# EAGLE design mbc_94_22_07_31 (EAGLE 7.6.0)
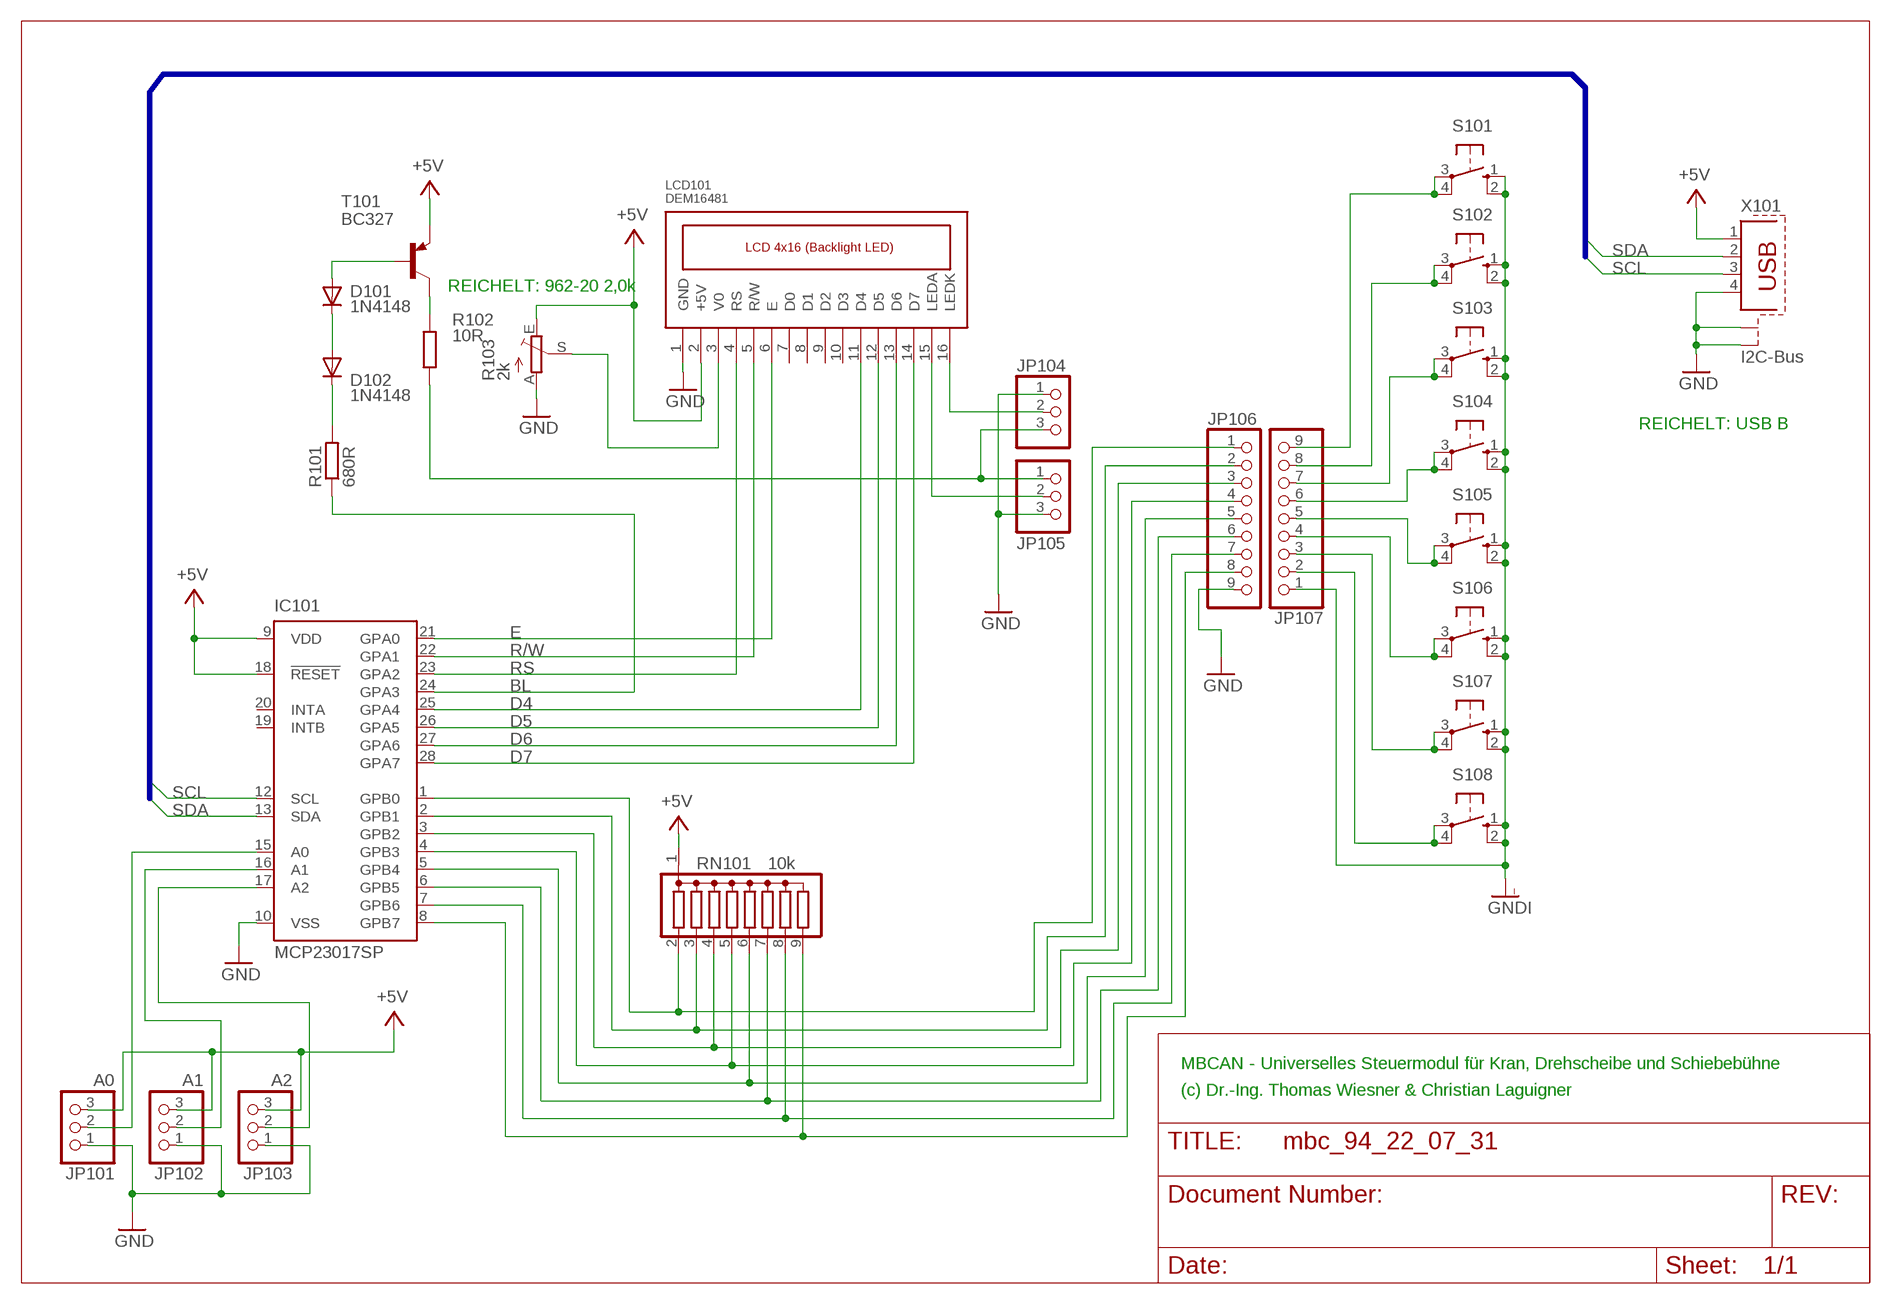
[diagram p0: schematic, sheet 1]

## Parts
D101  1N4148  1N4148DO35-10  [DO35-10]
D102  1N4148  1N4148DO35-10  [DO35-10]
IC101  MCP23017SP  [DIL28-3]
JP101  A0  PINHD-1X3  [1X03]
JP102  A1  PINHD-1X3  [1X03]
JP103  A2  PINHD-1X3  [1X03]
JP104  PINHD-1X3  [1X03]
JP105  PINHD-1X3  [1X03]
JP106  PINHD-1X9  [1X09]
JP107  PINHD-1X9  [1X09]
LCD101  DEM16481  [LCD4X16]
R101  680R  R-EU_0207/10  [0207/10]
R102  10R  R-EU_0207/10  [0207/10]
R103  2k  TRIM_EU-S43P  [SP19L]
RN101  10k  G08R  [SIL9]
S101  10-XX  [B3F-10XX]
S102  10-XX  [B3F-10XX]
S103  10-XX  [B3F-10XX]
S104  10-XX  [B3F-10XX]
S105  10-XX  [B3F-10XX]
S106  10-XX  [B3F-10XX]
S107  10-XX  [B3F-10XX]
S108  10-XX  [B3F-10XX]
T101  BC327  -PNP-TO92  [TO92]
X101  I2C-Bus  PN61729-S  [PN61729-S]

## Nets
+5V: IC101.9(VDD) IC101.18(!RESET) JP101.3 JP102.3 JP103.3 LCD101.2(+5V) R103.E RN101.1 T101.1(E) X101.1
BL: IC101.24(GPA3) R101.1
D4: IC101.25(GPA4) LCD101.11(D4)
D5: IC101.26(GPA5) LCD101.12(D5)
D6: IC101.27(GPA6) LCD101.13(D6)
D7: IC101.28(GPA7) LCD101.14(D7)
E: IC101.21(GPA0) LCD101.6(E)
GND: IC101.10(VSS) JP101.1 JP102.1 JP103.1 JP104.1 JP105.3 JP106.9 LCD101.1(GND) R103.A X101.4 X101.S1 X101.S2
GNDI: JP107.1 S101.1(S) S101.2(S1) S102.1(S) S102.2(S1) S103.1(S) S103.2(S1) S104.1(S) S104.2(S1) S105.1(S) S105.2(S1) S106.1(S) S106.2(S1) S107.1(S) S107.2(S1) S108.1(S) S108.2(S1)
N$1: IC101.1(GPB0) JP106.1 RN101.2
N$2: IC101.2(GPB1) JP106.2 RN101.3
N$3: IC101.3(GPB2) JP106.3 RN101.4
N$4: IC101.4(GPB3) JP106.4 RN101.5
N$5: IC101.5(GPB4) JP106.5 RN101.6
N$6: IC101.6(GPB5) JP106.6 RN101.7
N$7: IC101.7(GPB6) JP106.7 RN101.8
N$8: IC101.8(GPB7) JP106.8 RN101.9
N$11: JP105.2 LCD101.15(LEDA)
N$12: JP104.2 LCD101.16(LEDK)
N$14: JP107.9 S101.3(P) S101.4(P1)
N$15: JP107.8 S102.3(P) S102.4(P1)
N$16: JP107.7 S103.3(P) S103.4(P1)
N$17: JP107.6 S104.3(P) S104.4(P1)
N$18: JP107.5 S105.3(P) S105.4(P1)
N$19: JP107.4 S106.3(P) S106.4(P1)
N$20: JP107.3 S107.3(P) S107.4(P1)
N$21: JP107.2 S108.3(P) S108.4(P1)
N$22: IC101.15(A0) JP101.2
N$23: IC101.16(A1) JP102.2
N$24: LCD101.3(V0) R103.S
N$25: D102.C R101.2
N$26: D101.C D102.A
N$27: D101.A T101.2(B)
N$28: R102.2 T101.3(C)
N$29: IC101.17(A2) JP103.2
N$35: JP104.3 JP105.1 R102.1
R/W: IC101.22(GPA1) LCD101.5(R/W)
RS: IC101.23(GPA2) LCD101.4(RS)
SCL: IC101.12(SCL) X101.3
SDA: IC101.13(SDA) X101.2
Unconnected: IC101.19(INTB) IC101.20(INTA) LCD101.7(D0) LCD101.8(D1) LCD101.9(D2) LCD101.10(D3)

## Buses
B$3

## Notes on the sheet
- REICHELT: 962-20 2,0k
- REICHELT: USB B
- MBCAN - Universelles Steuermodul für Kran, Drehscheibe und Schiebebühne
- (c) Dr.-Ing. Thomas Wiesner & Christian Laguigner

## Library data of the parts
D101 D102 = diode:1N4148: DIODE
IC101 = microchip:MCP23017: http://ww1.microchip.com/downloads/en/DeviceDoc/21952a.pdf Source: http://ww1.microchip.com/downloads/en/DeviceDoc/21952a.pdf; MF: MICROCHIP; MPN: MCP23017-E/SP; OC_FARNELL: 1332088; OC_NEWARK: 31K2959
JP101-JP105 = pinhead:PINHD-1X3: PIN HEADER
JP106 JP107 = pinhead:PINHD-1X9: PIN HEADER
LCD101 = mbc:DEM16481
R101 R102 = resistor:R-EU_: RESISTOR, European symbol
R103 = pot:TRIM_EU-: POTENTIOMETER
RN101 = resistor-sil:G08R: SIL RESISTOR; OC_FARNELL: unknown; OC_NEWARK: unknown
S101-S108 = switch-omron:10-XX: OMRON SWITCH; MPN: B3F-1000; OC_FARNELL: 176432; OC_NEWARK: 36M3542
T101 = transistor:*-PNP-: PNP Transistror
X101 = con-berg:PN61729-S: BERG USB connector; OC_FARNELL: unknown; OC_NEWARK: unknown

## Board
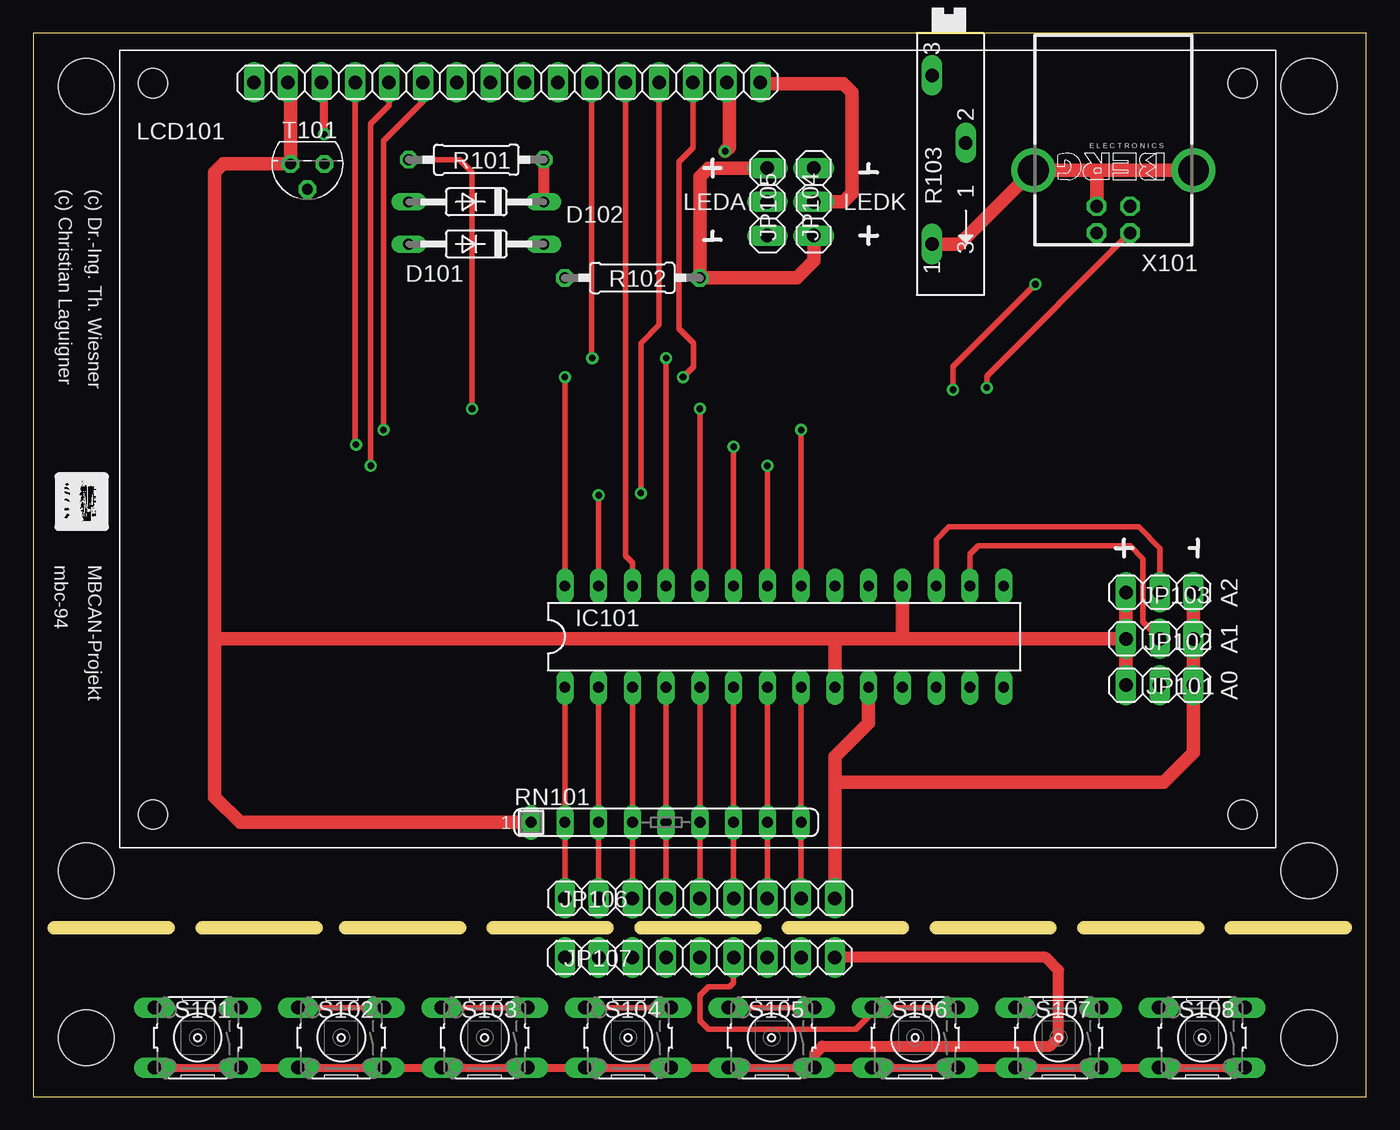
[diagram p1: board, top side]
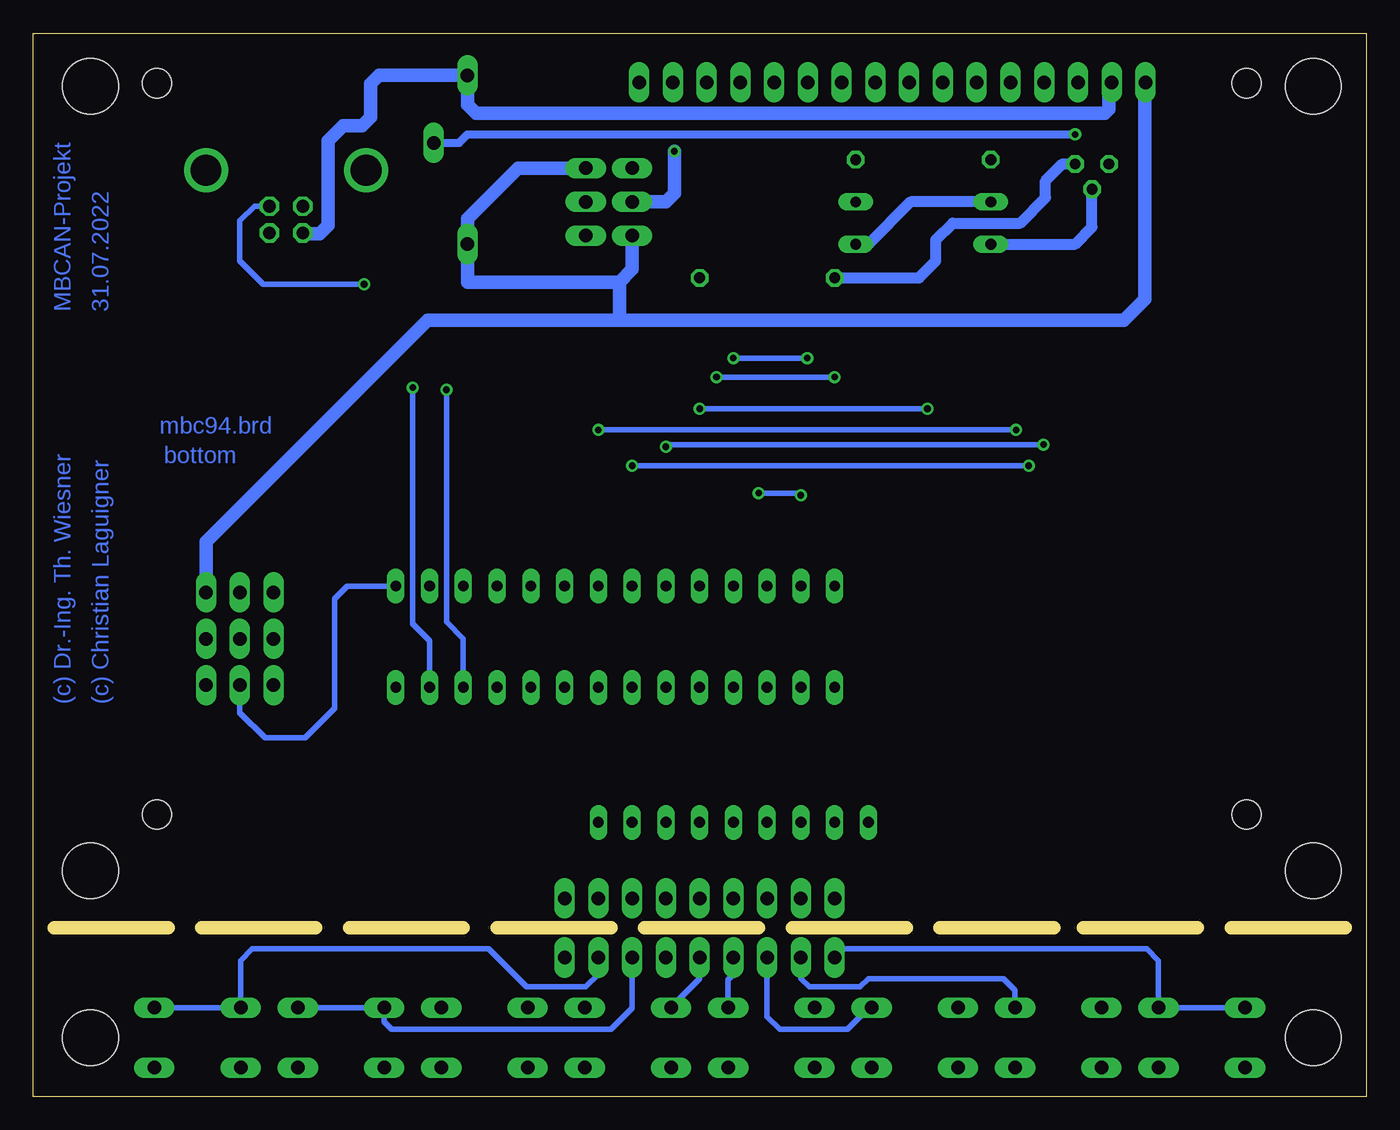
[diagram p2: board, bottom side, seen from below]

Size 100.31 x 80 mm. Coordinates in mm from the lower left corner, seen from the top.
Outline: 0,0 100.31,0 100.31,80 0,80 0,0
Copper layers (1*16): Top 0.035mm / dielectric 1.5mm / Bottom 0.035mm
Design rules "default *": minimum track width 10mil, minimum drill 0.5mm, track to track 8mil, track to pad 8mil, pad to pad 8mil, via to via 8mil, smd to smd 8mil, copper to edge 40mil, drill to drill 8mil, minimum pad ring 10mil, minimum via ring 8mil, stop-mask expansion 4mil, vias tented up to drill 0mil, thermal gap 10mil
Holes 4.2 mm at 4,76 96,76 4,4.45 96,4.45 4,17 96,17
Milling: 9 lines

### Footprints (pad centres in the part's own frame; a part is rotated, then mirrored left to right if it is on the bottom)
DO35-10 = drill 0.813 long: A 5.08,0; C -5.08,0
DIL28-3 = drill 0.813 long: 1 -16.51,-3.81; 2 -13.97,-3.81; 3 -11.43,-3.81; 4 -8.89,-3.81; 5 -6.35,-3.81; 6 -3.81,-3.81; 7 -1.27,-3.81; 8 1.27,-3.81; 9 3.81,-3.81; 10 6.35,-3.81; 11 8.89,-3.81; 12 11.43,-3.81; 13 13.97,-3.81; 14 16.51,-3.81; 15 16.51,3.81; 16 13.97,3.81; 17 11.43,3.81; 18 8.89,3.81; 19 6.35,3.81; 20 3.81,3.81; 21 1.27,3.81; 22 -1.27,3.81; 23 -3.81,3.81; 24 -6.35,3.81; 25 -8.89,3.81; 26 -11.43,3.81; 27 -13.97,3.81; 28 -16.51,3.81
1X03 = drill 1.016 long: 1 -2.54,0; 2 0,0; 3 2.54,0
1X09 = drill 1.016 long: 1 -10.16,0; 2 -7.62,0; 3 -5.08,0; 4 -2.54,0; 5 0,0; 6 2.54,0; 7 5.08,0; 8 7.62,0; 9 10.16,0
LCD4X16 = drill 1.016 long: 1 10.11,57.57; 2 12.65,57.57; 3 15.19,57.57; 4 17.73,57.57; 5 20.27,57.57; 6 22.81,57.57; 7 25.35,57.57; 8 27.89,57.57; 9 30.43,57.57; 10 32.97,57.57; 11 35.51,57.57; 12 38.05,57.57; 13 40.59,57.57; 14 43.13,57.57; 15 45.67,57.57; 16 48.21,57.57 | hole 2.2: 2.5,2.5; 2.5,57.5; 84.5,57.5; 84.5,2.5
0207/10 = drill 0.813 octagon: 1 -5.08,0; 2 5.08,0
SP19L = drill 1.016 long: A 5.715,-1.27; E -6.985,-1.27; S -1.905,1.27
SIL9 = drill 0.813 long: 1 -10.16,0; 2 -7.62,0; 3 -5.08,0; 4 -2.54,0; 5 0,0; 6 2.54,0; 7 5.08,0; 8 7.62,0; 9 10.16,0
B3F-10XX = drill 1.016 long: 1 -3.251,2.261; 2 3.251,2.261; 3 -3.251,-2.261; 4 3.251,-2.261
TO92 = drill 0.813 octagon: 1 1.27,0; 2 0,1.905; 3 -1.27,0
PN61729-S = drill 0.95 octagon: 1 1.25,4.71; 2 -1.25,4.71; 3 -1.25,2.71; 4 1.25,2.71 | drill 2.3 pad 2.9: S1 -6.02,0; S2 6.02,0

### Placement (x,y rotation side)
D101  33.34,64.14 180 top
D102  33.34,67.31 180 top
IC101  56.52,34.61 0 top
JP101  84.77,30.96 180 top
JP102  84.77,34.45 180 top
JP103  84.77,37.94 180 top
JP104  58.74,67.31 270 top
JP105  55.24,67.31 270 top
JP106  50.16,14.92 0 top
JP107  50.16,10.48 180 top
LCD101  6.51,18.73 0 top
R101  33.34,70.48 0 top
R102  45.09,61.59 180 top
R103  68.9,69.85 270 top
RN101  47.62,20.64 0 top
S101  12.38,4.45 180 top
S102  23.18,4.45 180 top
S103  33.97,4.45 180 top
S104  44.77,4.45 180 top
S105  55.56,4.45 180 top
S106  66.36,4.45 180 top
S107  77.15,4.45 180 top
S108  87.95,4.45 180 top
T101  20.64,70.17 180 top
X101  81.28,69.69 180 top

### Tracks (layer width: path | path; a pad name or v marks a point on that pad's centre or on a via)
+5V
  Top 1.016: RN101.1 15.56,20.64 13.65,22.54 13.65,34.45 | 13.65,34.45 13.65,69.53 14.29,70.17 T101.1 19.37,76.25 LCD101.2 | IC101.9 60.33,34.45 | 60.33,34.45 13.65,34.45 | 60.33,34.45 65.41,34.45 | JP103.3 JP102.3 | JP102.3 JP101.3 | IC101.18 65.41,34.45 | 65.41,34.45 JP102.3
  Bottom 1.016: LCD101.2 19.37,76.25 19.37,74.3 19.68,73.98 66.99,73.98 67.63,74.61 R103.E 74.3,76.83 74.93,76.2 74.93,73.66 75.56,73.03 76.99,73.03 78.11,71.91 78.11,65.56 78.74,64.93 79.98,64.93 X101.1
BL  (via drill 0.5)
  Top 0.406: v33.02,51.75 33.02,69.53 32.07,70.48 R101.1 | v50.16,51.75 IC101.24
  Bottom 0.406: v33.02,51.75 v50.16,51.75
D4  (via drill 0.5)
  Top 0.406: LCD101.11 42.02,55.61 v42.07,55.56 | v47.62,55.56 IC101.25
  Bottom 0.406: v42.07,55.56 v47.62,55.56
D5
  Top 0.406: LCD101.12 44.56,40.69 45.09,40.16 IC101.26
D6  (via drill 0.5)
  Top 0.406: LCD101.13 47.1,58.05 45.72,56.67 v45.72,45.4 | v42.55,45.24 IC101.27
  Bottom 0.406: v45.72,45.4 42.7,45.4 v42.55,45.24
D7  (via drill 0.5)
  Top 0.406: LCD101.14 49.64,71.39 48.58,70.33 48.58,57.78 49.69,56.67 49.69,54.93 v48.9,54.13 | v40.01,54.13 IC101.28
  Bottom 0.406: v48.9,54.13 v40.01,54.13
E  (via drill 0.5)
  Top 0.406: LCD101.6 29.32,74.88 26.35,71.91 v26.35,50.16 | v57.78,50.16 IC101.21
  Bottom 0.406: v26.35,50.16 v57.78,50.16
GND
  Top 1.016: X101.S1 80.17,69.69 | 80.17,69.69 X101.S2 75.25,69.69 69.69,64.14 R103.A | X101.4 80.03,69.55 80.17,69.69 | JP106.9 60.33,23.65 | 60.33,23.65 60.33,25.56 62.87,28.1 IC101.10 | JP103.1 JP102.1 JP101.1 87.31,25.88 85.09,23.65 60.33,23.65
  Bottom 1.016: LCD101.1 16.68,76.2 16.68,60 18.26,58.42 56.2,58.42 | JP104.1 63.82,69.85 67.63,66.04 R103.A 67.63,61.28 56.2,61.28 | JP105.3 55.24,62.23 56.2,61.28 | 56.2,58.42 56.2,61.28 | 56.2,58.42 70.64,58.42 87.31,41.75 JP103.1
GNDI
  Top 0.61: S101.2 S101.1 S102.2 S102.1 S103.2 S103.1 S104.2 S104.1 S105.2 58.42,2.18 58.42,2.22 58.81,2.22 S105.1 S106.2 S106.1 S107.2 S107.1 S108.2 S108.1
  Top 0.813: 58.81,2.22 58.81,3.25 59.37,3.81 76.52,3.81 77.15,4.45 77.15,9.53 76.2,10.48 JP107.1
N$1
  Top 0.406: JP106.1 RN101.2 IC101.1
N$2
  Top 0.406: JP106.2 RN101.3 IC101.2
N$3
  Top 0.406: JP106.3 RN101.4 IC101.3
N$4
  Top 0.406: JP106.4 RN101.5 IC101.4
N$5
  Top 0.406: JP106.5 RN101.6 IC101.5
N$6
  Top 0.406: JP106.6 RN101.7 IC101.6
N$7
  Top 0.406: JP106.7 RN101.8 IC101.7
N$8
  Top 0.406: JP106.8 RN101.9 IC101.8
N$11  (via drill 0.5)
  Top 1.016: v52.07,71.12 52.39,71.44 52.39,76.25 LCD101.15
  Bottom 1.016: JP105.2 52.7,67.31 52.07,67.94 v52.07,71.12
N$12
  Top 1.016: JP104.2 60.96,67.31 61.59,67.94 61.59,75.56 60.96,76.2 54.98,76.2 LCD101.16
N$14
  Bottom 0.406: S101.4 S101.3 15.63,10.24 16.51,11.11 39.37,11.11 JP107.9
N$15
  Top 0.406: S102.4 S102.3
  Bottom 0.406: S102.3 26.43,8.01 27.3,8.89 37.47,8.89 38.1,8.26 41.91,8.26 42.55,8.89 JP107.8
N$16
  Top 0.406: S103.4 S103.3
  Bottom 0.406: S103.3 37.43,6.71 39.05,5.08 44.13,5.08 45.09,6.03 JP107.7
N$17
  Top 0.406: S104.4 S104.3
  Bottom 0.406: S104.3 48.02,8.81 47.62,9.21 JP107.6
N$18
  Top 0.406: S105.4 S105.3
  Bottom 0.406: S105.4 52.31,6.74 50.16,8.89 JP107.5
N$19
  Top 0.406: S106.3 S106.4 63.11,6.27 61.91,5.08 50.8,5.08 50.16,5.71 50.16,7.62 50.8,8.26 52.39,8.26 52.7,8.57 JP107.4
N$20
  Bottom 0.406: S107.3 S107.4 73.9,5.64 73.34,5.08 56.83,5.08 55.24,6.67 JP107.3
N$21
  Bottom 0.406: S108.3 S108.4 84.7,10.24 83.82,11.11 66.04,11.11 63.18,8.26 58.74,8.26 57.78,9.21 JP107.2
N$22
  Bottom 0.406: IC101.15 76.68,38.42 77.63,37.47 77.63,29.21 79.85,26.99 82.87,26.99 84.77,28.89 JP101.2
N$23
  Top 0.406: IC101.16 70.48,40.8 71.12,41.43 82.55,41.43 83.5,40.48 83.5,35.72 JP102.2
N$24  (via drill 0.5)
  Top 0.61: v21.91,72.39 21.91,76.25 LCD101.3
  Bottom 0.61: R103.S 68.26,71.75 67.63,72.39 v21.91,72.39
N$25
  Top 0.813: R101.2 D102.C
N$26
  Bottom 0.813: D102.A 34.29,67.31 37.47,64.14 D101.C
N$27
  Bottom 0.813: D101.A 21.91,64.14 20.64,65.41 T101.2
N$28
  Bottom 0.813: R102.2 33.66,61.59 32.38,62.87 32.38,64.45 31.11,65.72 26.04,65.72 24.13,67.63 24.13,68.9 22.86,70.17 T101.3
N$29
  Top 0.406: IC101.17 67.94,41.91 68.9,42.86 83.19,42.86 84.77,41.27 JP103.2
N$35
  Top 1.016: JP104.3 58.74,62.87 57.47,61.59 R102.1 50.16,69.22 50.8,69.85 JP105.1
R/W  (via drill 0.5)
  Top 0.406: LCD101.5 26.78,74.56 25.4,73.18 v25.4,47.47 | v55.24,47.47 55.24,39.05 55.4,38.89 55.4,38.58 IC101.22
  Bottom 0.406: v25.4,47.47 v55.24,47.47
RS  (via drill 0.5)
  Top 0.406: LCD101.4 24.24,49.1 v24.29,49.05 | v52.7,48.9 IC101.23
  Bottom 0.406: v24.29,49.05 52.55,49.05 v52.7,48.9
SCL  (via drill 0.5)
  Top 0.406: v69.22,53.18 69.22,54.93 v75.41,61.12
  Bottom 0.406: IC101.12 67.94,34.45 69.22,35.72 v69.22,53.18 | v75.41,61.12 83.03,61.12 84.77,62.87 84.77,65.88 83.66,66.99 82.54,66.99 X101.3
SDA  (via drill 0.5)
  Top 0.406: v71.75,53.34 71.75,54.21 X101.2
  Bottom 0.406: IC101.13 70.48,34.29 71.75,35.56 v71.75,53.34

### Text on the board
Bottom: 31.07.2022 | MBCAN-Projekt | mbc94.brd | bottom | (c) Christian Laguigner | (c) Dr.-Ing. Th. Wiesner
tNames: (c) Christian Laguigner | (c) Dr.-Ing. Th. Wiesner | LEDA | LEDK | mbc-94 | MBCAN-Projekt | A2 | A1 | A0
